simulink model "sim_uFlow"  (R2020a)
settings: Solver=ode4  StartTime=0.0  StopTime=tsim  FixedStep=1  MaxStep=1  RelTol=1e-8
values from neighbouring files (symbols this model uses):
  dnom = [T0nom; TDnom; qDnom; Qnom]    [runTransformedMVs.m]
  Kc = 1./(tauC+theta)    [runTransformedMVs.m]
  KcS = 1/kuv*tuv/(tauCS+thetauv)    (= -0.000668553381732)    [runTransformedMVs.m]
  p = [V1;V2;rho;cp;A1;A2;tau01; tau02;transf]    [runTransformedMVs.m]
  T2nom = 30    [runTransformedMVs.m]
  tauI = 4.*(tauC+theta)    [runTransformedMVs.m]
  tauIS = min(tuv,4*(tauCS+thetauv))    [runTransformedMVs.m]
  Tnom = [T1nom;T2nom]    [runTransformedMVs.m]
  ubias = Qnom    (= 1672)    [runTransformedMVs.m]
  umax = 3*Qnom    (= 5016)    [runTransformedMVs.m]
  umin = 1e-4    (= 0.0001)    [runTransformedMVs.m]
  vbias = [0;0]    [runTransformedMVs.m]
undefined symbols (not defined in the file or in its folder): CalcBlock_v, Tank

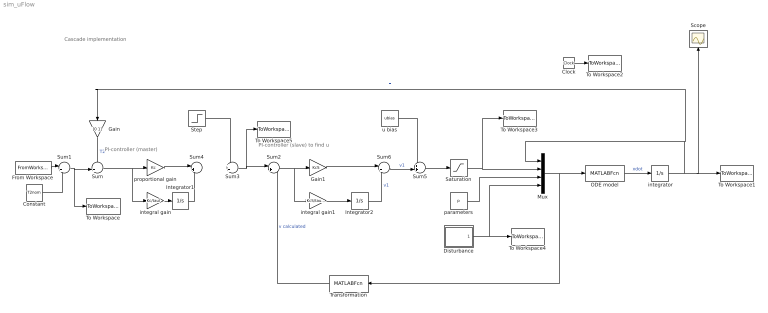
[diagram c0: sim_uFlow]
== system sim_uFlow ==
  note: Cascade implementation
  note: PI-controller (master)
  note: PI-controller (slave) to find u
  " integrator" : Integrator  InitialCondition=Tnom
  Clock : Clock
  Constant : Constant  Value=T2nom
  Disturbance : Subsystem
  From Workspace : FromWorkspace  VariableName=T2sp  OutputAfterFinalValue=Holding final value
  Gain : Gain  Gain=[0 1]  Multiplication=Matrix(K*u)
  Gain1 : Gain  Gain=KcS  Multiplication=Matrix(K*u)
  Integrator1 : Integrator
  Integrator2 : Integrator
  Mux : Mux
  ODE model : MATLABFcn  MATLABFcn=Tank(u(1:2), u(3),u(4:12),u(13:16))  OutputDimensions=2
  Saturation : Saturate  UpperLimit=umax  LowerLimit=umin
  Scope : Scope
  Step : Step  Time=1000  Before=vbias  After=vbias*0.1  SampleTime=0
  Sum : Sum  Inputs=-+|
  Sum1 : Sum  Inputs=|++
  Sum2 : Sum  Inputs=|+-
  Sum3 : Sum  Inputs=++|
  Sum4 : Sum  Inputs=|++
  Sum5 : Sum  Inputs=++|
  Sum6 : Sum  Inputs=|++
  To Workspace : ToWorkspace  VariableName=Tsp  SampleTime=-1
  To Workspace1 : ToWorkspace  VariableName=T  SampleTime=-1
  To Workspace2 : ToWorkspace  VariableName=time  SampleTime=-1
  To Workspace3 : ToWorkspace  VariableName=u  SampleTime=-1
  To Workspace4 : ToWorkspace  VariableName=d  SampleTime=-1
  To Workspace5 : ToWorkspace  VariableName=vsp  SampleTime=-1
  Transformation : MATLABFcn  MATLABFcn=CalcBlock_v(u(1:2), u(3),u(4:12),u(13:16))  OutputDimensions=1
  integral gain : Gain  Gain=Kc/tauI  Multiplication=Matrix(K*u)
  integral gain1 : Gain  Gain=KcS/tauIS  Multiplication=Matrix(K*u)
  parameters : Constant  Value=p
  proportional gain : Gain  Gain=Kc  Multiplication=Matrix(K*u)
  u bias : Constant  Value=ubias
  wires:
  " integrator"/1 -> To Workspace1/1, Scope/1, Mux/1, Gain/1  "T"
  Mux/1 -> Transformation/1, ODE model/1
  Clock/1 -> To Workspace2/1
  Sum5/1 -> Saturation/1
  ODE model/1 -> " integrator"/1  "xdot"
  parameters/1 -> Mux/3
  Saturation/1 -> Mux/2, To Workspace3/1
  Disturbance/1(d) -> To Workspace4/1, Mux/4
  Sum1/1 -> Sum/2, To Workspace/1
  Gain/1 -> Sum/1  "T2"
  From Workspace/1 -> Sum1/1
  Constant/1 -> Sum1/2
  Sum3/1 -> Sum2/1, To Workspace5/1
  Sum/1 -> integral gain/1, proportional gain/1
  Integrator1/1 -> Sum4/2
  Step/1 -> Sum3/1
  integral gain/1 -> Integrator1/1
  proportional gain/1 -> Sum4/1
  Sum4/1 -> ?  "v2"
  Sum6/1 -> Sum5/2  "v1"
  Sum2/1 -> Gain1/1, integral gain1/1
  u bias/1 -> Sum5/1
  integral gain1/1 -> Integrator2/1
  Transformation/1 -> Sum2/2  "v calculated"
  Gain1/1 -> Sum6/1
  Integrator2/1 -> Sum6/2  "v1"

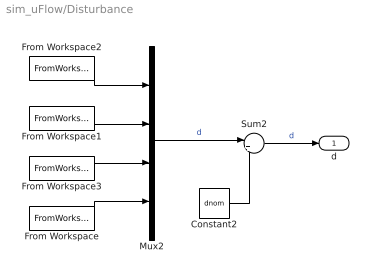
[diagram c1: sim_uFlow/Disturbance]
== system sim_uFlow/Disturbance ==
  Constant2 : Constant  Value=dnom
  From Workspace : FromWorkspace  VariableName=dist{4}  OutputAfterFinalValue=Setting to zero
  From Workspace1 : FromWorkspace  VariableName=dist{2}  OutputAfterFinalValue=Setting to zero
  From Workspace2 : FromWorkspace  VariableName=dist{1}  OutputAfterFinalValue=Setting to zero
  From Workspace3 : FromWorkspace  VariableName=dist{3}  OutputAfterFinalValue=Setting to zero
  Mux2 : Mux
  Sum2 : Sum  Inputs=|++
  d : Outport
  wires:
  From Workspace2/1 -> Mux2/1
  From Workspace/1 -> Mux2/4
  From Workspace3/1 -> Mux2/3
  Mux2/1 -> Sum2/1  "d"
  Constant2/1 -> Sum2/2
  From Workspace1/1 -> Mux2/2
  Sum2/1 -> d/1  "d"
